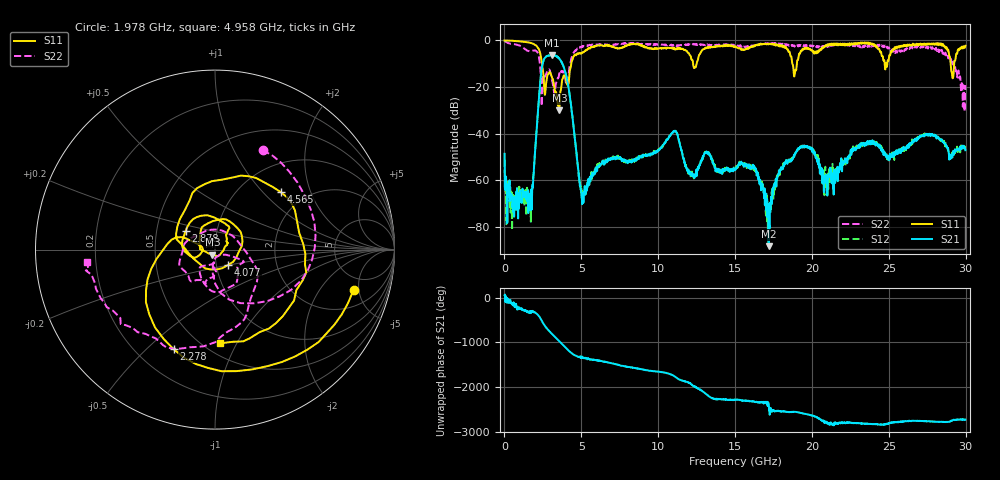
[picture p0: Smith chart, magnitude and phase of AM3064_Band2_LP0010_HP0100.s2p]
# Hz S DB R 50.0
!freq dBS11 angS11 dBS21 angS21 dBS12 angS12 dBS22 angS22
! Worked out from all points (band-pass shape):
!   1600 points, 10 MHz to 29.98 GHz, reference 50 ohm
!   highest |S21| = -6.27 dB at 3.065 GHz (marker M1); lowest = -88.2 dB at 17.18 GHz (marker M2)
!   |S21| within 3 dB of the highest: 2.512 GHz to 3.714 GHz (1.203 GHz wide, 38.6 % of centre)
!   lowest |S11| = -29.9 dB at 3.571 GHz (marker M3), VSWR 1.07, Z = 48.5 - j2.75 ohm
!   |S11| at or under -10 dB: 2.435 GHz to 4.344 GHz (1.909 GHz wide, 56.3 % of centre); 12.27 GHz to 12.5 GHz (229.7 MHz wide, 1.86 % of centre); 18.73 GHz to 19.02 GHz (291.9 MHz wide, 1.55 % of centre)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
!   |S22| runs from -30.5 to -0.2 dB; largest |S21 - S12| = 0.012
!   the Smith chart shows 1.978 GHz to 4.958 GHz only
!   S11 on the Smith chart (normalised r, x): 1.978 GHz: 3.45, -4.40; 2.278 GHz: 0.35, -0.61; 2.878 GHz: 0.71, +0.15; 4.077 GHz: 1.14, -0.20; 4.565 GHz: 1.52, +1.27; 4.958 GHz: 0.60, -0.86
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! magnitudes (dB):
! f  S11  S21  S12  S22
! 10 MHz  0.0  -48.6  -51.0  -0.2
! 1.641 GHz  -1.0  -69.7  -71.3  -4.7
! 1.978 GHz  -1.9  -48.6  -48.8  -4.2
! 2.278 GHz  -4.4  -21.6  -21.6  -8.6
! 2.878 GHz  -14.3  -6.5  -6.5  -12.5
! 3.065 GHz  -15.5  -6.3  -6.2  -16.1
! 3.571 GHz  -29.9  -7.9  -7.8  -14.1
! 4.077 GHz  -19.0  -16.9  -17.0  -18.9
! 4.565 GHz  -6.2  -41.3  -41.2  -4.5
! 4.958 GHz  -5.6  -64.0  -63.1  -2.9
! 5.015 GHz  -5.6  -67.5  -63.2  -3.0
! 10 GHz  -3.5  -47.2  -46.7  -1.8
! 15 GHz  -2.5  -54.9  -54.8  -1.9
! 16.28 GHz  -2.2  -54.9  -54.2  -2.1
! 17.18 GHz  -1.7  -88.2  -74.3  -1.6
! 18.23 GHz  -3.2  -52.2  -53.0  -1.6
! 19.99 GHz  -4.1  -46.4  -46.5  -2.2
! 20.91 GHz  -2.1  -59.3  -58.7  -2.4
! 25 GHz  -8.2  -51.1  -49.8  -3.0
! 28.56 GHz  -2.1  -43.7  -43.1  -4.7
! 29.16 GHz  -16.2  -48.6  -49.2  -8.8
! 29.98 GHz  -2.3  -47.0  -46.6  -19.2
